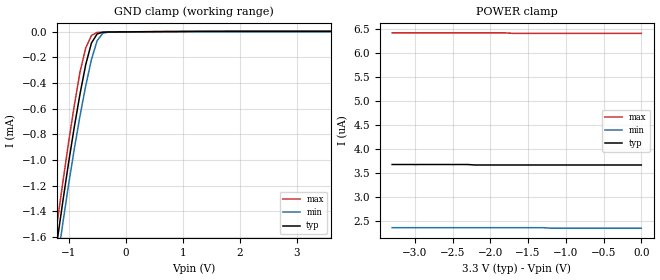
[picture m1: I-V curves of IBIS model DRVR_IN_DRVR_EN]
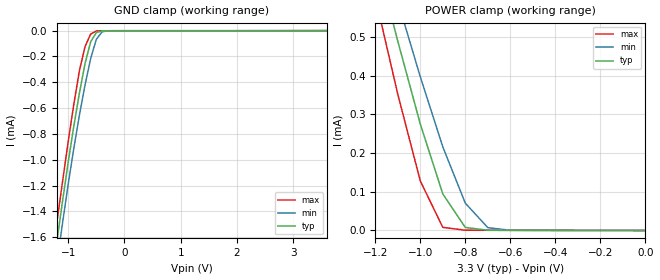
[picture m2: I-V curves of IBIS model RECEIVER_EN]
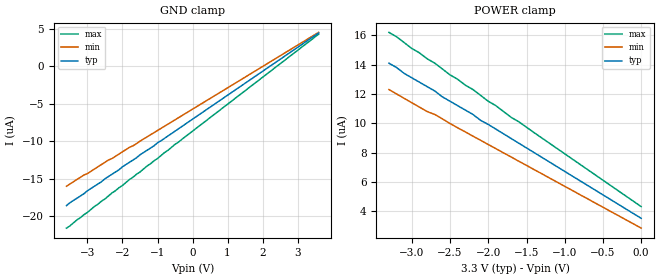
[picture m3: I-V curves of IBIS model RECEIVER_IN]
|   Texas Instruments Incorporated
|   Data Transmissions Products
|   IBIS Model for SN65MLVD205
|   14D SOIC Package
[IBIS Ver]   3.2
[Comment char]   |_char
[File name]   mlvd205.ibs
[File Rev]   2.0
[Date]   15Apr02
[Source]   File originated at Texas Instruments Incorporated.
   Data Transmission Products Group. All data based on
   Bench Measurements.
[Notes]   This model was revved in Aug03 to correct for Vod  -TMF-
   This model was revved in Aug03 to add min and max.
[Disclaimer]
(C) Copyright Texas Instruments Incorporated 2003
   All rights reserved
  Texas Instruments Incorporated hereby grants the user of this IBIS
model a non-exclusive, nontransferable license to use this IBIS model
under the following terms.  Before using this IBIS model, the user
should read this license.  If the user does not accept these terms,
the IBIS model should be returned to Texas Instruments within 30 days.
  The user is granted this license only to use the IBIS model and
is not granted rights to sell, load, rent, lease or license the IBIS
model in whole or in part, or in modified form to anyone other than
user.  User may modify the IBIS model to suit its specific applications
but rights to derivative works and such modifications shall belong to
Texas Instruments.
  This IBIS model is provided on an "AS IS" basis and Texas Instruments
makes absolutely no warranty with respect to the information contained
herein.  TEXAS INSTRUMENTS DISCLAIMS AND CUSTOMER WAIVES ALL WARRANTIES,
EXPRESS OR IMPLIED, INCLUDING WARRANTIES OF MERCHANTABILITY OR FITNESS
FOR A PARTICULAR PURPOSE. The entire risk as to quality and performance
is with the Customer. ACCORDINGLY, IN NO EVENT SHALL THE COMPANY BE LIABLE
FOR ANY DAMAGES, WHETHER IN CONTRACT OR TORT,INCLUDING ANY LOST PROFITS
OR OTHER INCIDENTAL, CONSEQUENTIAL, EXEMPLARY, OR PUNITIVE DAMAGES ARISING
OUT OF THE USE OR APPLICATION OF THE IBIS model provided in this package.
Further, Texas Instruments reserves the right to discontinue or make changes
without notice to any product herein to improve reliability, function, or
design. Texas Instruments does not convey any license under patent rights
or any other intellectual property rights, including those of third parties.
Contact Texas Instruments at ATTN:DATA TRANSMISSIONS
[Copyright]   Copyright 2003, Texas Instruments, All Rights Reserved
[Component]   SN65MLVD205D
[Manufacturer]  Texas Instruments Incorporated
[Package]
|   typ   min   max
R_pkg   0.031   0.028   0.034
L_pkg   3.109nH   2.462nH   3.889nH
C_pkg   0.473pF   0.363pF   0.628pF
[Pin]   signal_name   model_name   R_pin   L_pin   C_pin
1   NC   NC
2   R   RECEIVER_OUT   0.032   3.188n   0.473p
3   RE   RECEIVER_EN   0.028   2.462n   0.377p
4   DE   DRVR_IN_DRVR_EN   0.031   2.596n   0.363p
5   D   DRVR_IN_DRVR_EN   0.028   2.521n   0.372p
6   GND   GND   0.034   3.250n   0.476p
7   GND   GND   0.034   3.889n   0.628p
8   NC   NC
9   Y   DRIVER_OUT   0.034   3.250n   0.476p
10   Z   DRIVER_OUT   0.028   2.521n   0.372p
11   B   RECEIVER_IN   0.031   2.596n   0.364p
12   A   RECEIVER_IN   0.028   2.462n   0.377p
13   VCC   POWER   0.032   3.188n   0.473p
14   VCC   POWER   0.033   3.854n   0.622p
[Diff_pin]   inv_pin   vdiff   tdelay_typ   tdelay_min   tdelay_max
| The 'A' or 'Y' pins are Diff_pins and the 'B' or 'Z' pins are inv_pins
   12   11   0.05   0   0   0
   9   10   0.00   0   0   0
| Models and submodels in the file (5): DRVR_IN_DRVR_EN (Input), RECEIVER_EN (Input), RECEIVER_IN (Input), DRIVER_OUT (3-state), RECEIVER_OUT (3-state)
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|   Driver/Driver Enable Model
[Model]   DRVR_IN_DRVR_EN
Model_type   Input
|Signals   D,DE
Vinh = 2.0
Vinl = 0.8
|   typ   min   max
C_comp   3.59pF   3.46pF   3.65pF
|   typ   min   max
[Temperature Range]   25.0   85   -40
[Voltage range]   3.3V   3.0V   3.6V
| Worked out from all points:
|   GND clamp passes 1 mA (typ) near -0.99 V on its own axis
[GND_clamp]
|   Voltage   I(typ)   I(min)   I(max)
-3.6V     -11.3mA    -10.8mA    -12mA
-1.3V     -1.97mA    -2.12mA    -1.82mA
-1.2V     -1.63mA    -1.8mA     -1.49mA
-1.1V     -1.32mA    -1.49mA    -1.17mA
-900mV    -741uA     -913uA     -573uA
-800mV    -484uA     -655uA     -312uA
-700mV    -255uA     -420uA     -125uA
-600mV    -86.9uA    -216uA     -28.5uA
-500mV    -15.9uA    -68.4uA    -4.3uA
-400mV    -2.37uA    -10.5uA    -2.39uA
-300mV    -1.1uA     -1.5uA     -1.75uA
3.6V      3.66uA     2.34uA     6.41uA
[Power_clamp]
| Note that the[POWER_clamp]voltage table is referenced to Vcc
| and is calculated using Vtable=Vcc - Vmeasured.
|   Voltage   I(typ)   I(min)   I(max)
-3.3V     3.67uA     2.35uA     6.42uA
-2.3V     3.67uA     2.35uA     6.42uA
-2.2V     3.66uA     2.35uA     6.42uA
-1.8V     3.66uA     2.35uA     6.42uA
-1.7V     3.66uA     2.35uA     6.41uA
-1.3V     3.66uA     2.35uA     6.41uA
-1.2V     3.66uA     2.34uA     6.41uA
0V        3.66uA     2.34uA     6.41uA
|   Receiver Enable Model
[Model]   RECEIVER_EN
Model_type   Input
|Signals   RE
Vinh = 2.0
Vinl = 0.8
|   typ   min   max
C_comp   3.57pF   3.41pF   3.65pF
|   typ   min   max
[Temperature Range]   25.0   85   -40
[Voltage range]   3.3V   3.0V   3.6V
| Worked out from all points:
|   GND clamp passes 1 mA (typ) near -0.99 V on its own axis
|   POWER clamp passes 1 mA (typ) near -1.32 V on its own axis
[GND_clamp]
|   Voltage   I(typ)   I(min)   I(max)
-3.6V     -11.3mA    -10.8mA    -12mA
-1.3V     -1.97mA    -2.12mA    -1.82mA
-1.2V     -1.63mA    -1.8mA     -1.48mA
-1.1V     -1.32mA    -1.49mA    -1.17mA
-900mV    -740uA     -912uA     -571uA
-800mV    -483uA     -654uA     -310uA
-700mV    -254uA     -420uA     -123uA
-600mV    -86uA      -216uA     -26.3uA
-500mV    -14.9uA    -67.8uA    -2.14uA
-400mV    -1.52uA    -9.95uA    -835nA
-300mV    -611nA     -1.2uA     -813nA
3.6V      162nA      579nA      58.4pA
[Power_clamp]
| Note that the[POWER_clamp]voltage table is referenced to Vcc
| and is calculated using Vtable=Vcc - Vmeasured.
|   Voltage   I(typ)   I(min)   I(max)
-3.3V     5.83mA     5.34mA     6.38mA
-1.2V     714uA      795uA      603uA
-1.1V     489uA      592uA      352uA
-1V       275uA      397uA      128uA
-900mV    94.4uA     216uA      8.04uA
-800mV    7.83uA     70.6uA     640nA
-700mV    564nA      7.25uA     507nA
-600mV    340nA      579nA      432nA
0V        60pA       852pA      58.4pA
|   Receiver Input Model
[Model]   RECEIVER_IN
Model_type   Input
|Signals   A,B
Vinl = 1.15V
Vinh = 1.35V
|   typ   min   max
C_comp   3.06pF   3.05pF   3.11pF
|   typ   min   max
[Temperature Range]   25.0   85   -40
[Voltage range]   3.3V   3.0V   3.6V
[GND_clamp]
|   Voltage   I(typ)   I(min)   I(max)
-3.6V     -18.6uA    -16uA      -21.6uA
-3.5V     -18.2uA    -15.7uA    -21.3uA
-3.3V     -17.6uA    -15.1uA    -20.5uA
-3V       -16.6uA    -14.3uA    -19.5uA
-2.4V     -14.7uA    -12.5uA    -17.3uA
-1.7V     -12.5uA    -10.6uA    -14.8uA
3.6V      4.48uA     4.56uA     4.32uA
[Power_clamp]
| Note that the[POWER_clamp]voltage table is referenced to Vcc
| and is calculated using Vtable=Vcc - Vmeasured.
|   Voltage   I(typ)   I(min)   I(max)
-3.3V     14.1uA     12.3uA     16.2uA
-3.2V     13.8uA     12uA       15.9uA
-3.1V     13.4uA     11.7uA     15.5uA
-2.8V     12.5uA     10.8uA     14.4uA
-2.7V     12.2uA     10.6uA     14.1uA
-2.6V     11.8uA     10.3uA     13.7uA
-2.5V     11.5uA     9.98uA     13.3uA
-2.2V     10.6uA     9.12uA     12.3uA
-2.1V     10.2uA     8.84uA     11.9uA
-1.7V     8.96uA     7.7uA      10.4uA
-1.6V     8.64uA     7.41uA     10.1uA
0V        3.52uA     2.85uA     4.32uA
